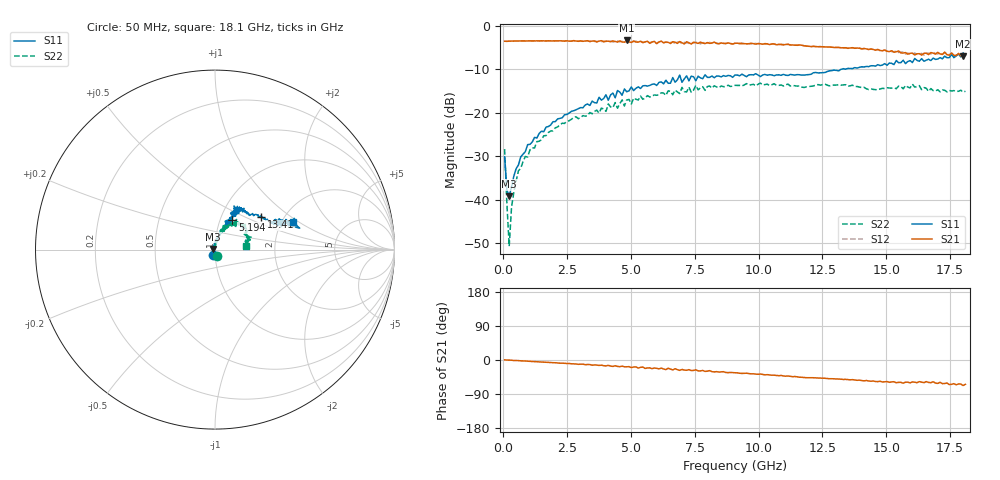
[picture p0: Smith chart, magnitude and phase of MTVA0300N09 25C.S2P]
! Network Analyzer HP8720D.06.14 Serial No. US36140669
! 28 Jun 2005  09:07:15
! Frequency  S11  S21  S12  S22
# HZ  S  DB R 50
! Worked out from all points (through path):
!   201 points, 50 MHz to 18.1 GHz, reference 50 ohm
!   highest |S21| = -3.39 dB at 4.833 GHz (marker M1); lowest = -6.9 dB at 18.01 GHz (marker M2)
!   group delay of S21, straight-line fit = 10.4 ps
!   lowest |S11| = -39.2 dB at 230.5 MHz (marker M3), VSWR 1.02, Z = 49 + j0.309 ohm
!   |S11| at or under -10 dB: start of sweep to 13.25 GHz; 13.40276 GHz to 13.40962 GHz (6.869 MHz wide, 0.0512 % of centre)
!   |S22| runs from -50.6 to -13.2 dB; largest |S21 - S12| = 0.038
!   S11 on the Smith chart (normalised r, x): 50 MHz: 0.98, -0.06; 5.194 GHz: 1.14, +0.39; 13.41 GHz: 1.55, +0.62; 18.1 GHz: 2.30, +0.89
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5e7  -30.09 -105.9  -3.57 0.4  -3.57 0.6  -28.36 -72.3
1.4025e8  -37.76 -150.4  -3.59 -0.1  -3.59 -0.1  -40.99 -112.9
2.305e8  -39.17 163.3  -3.55 -0.3  -3.54 -0.3  -50.64 170.6
3.2075e8  -37.06 131.1  -3.53 -0.5  -3.55 -0.5  -41.74 102.3
4.11e8  -34.57 113.7  -3.53 -1.2  -3.53 -1.2  -38.29 96.8
5.915e8  -31.98 100.0  -3.52 -1.6  -3.54 -1.7  -33.32 88.6
8.6225e8  -28.92 87.9  -3.52 -2.7  -3.52 -2.8  -30.05 87.9
1.94525e9  -22.05 75.1  -3.50 -7.1  -3.51 -7.0  -24.15 75.0
3.1185e9  -18.86 69.0  -3.58 -10.9  -3.60 -11.3  -20.66 74.0
4.83325e9  -15.18 68.3  -3.40 -18.0  -3.68 -18.6  -17.05 60.7
5.19425e9  -14.38 59.7  -3.75 -18.2  -3.56 -18.8  -16.91 68.9
6.09675e9  -13.03 60.9  -3.77 -23.4  -3.67 -23.1  -15.85 59.0
6.7285e9  -12.99 66.5  -3.80 -23.0  -4.10 -24.0  -14.80 52.4
6.909e9  -11.34 62.7  -3.65 -27.3  -3.74 -25.3  -15.59 52.2
6.99925e9  -13.00 62.9  -3.93 -24.9  -4.14 -27.1  -14.18 52.8
7.17975e9  -11.52 66.4  -3.68 -27.1  -3.96 -25.3  -15.23 48.0
9.075e9  -11.33 58.1  -4.04 -33.7  -4.01 -33.9  -13.70 43.3
1.21435e10  -10.81 43.6  -4.76 -46.8  -4.72 -47.0  -13.85 39.6
1.3407e10  -10.01 35.0  -5.09 -51.1  -5.07 -51.6  -13.56 32.7
1.512175e10  -8.58 23.1  -5.95 -58.9  -5.71 -58.5  -14.32 25.5
1.800975e10  -6.25 14.2  -6.93 -67.3  -6.73 -67.0  -15.28 12.2
1.81e10  -6.73 19.3  -6.78 -64.2  -7.06 -64.8  -15.06 7.1
